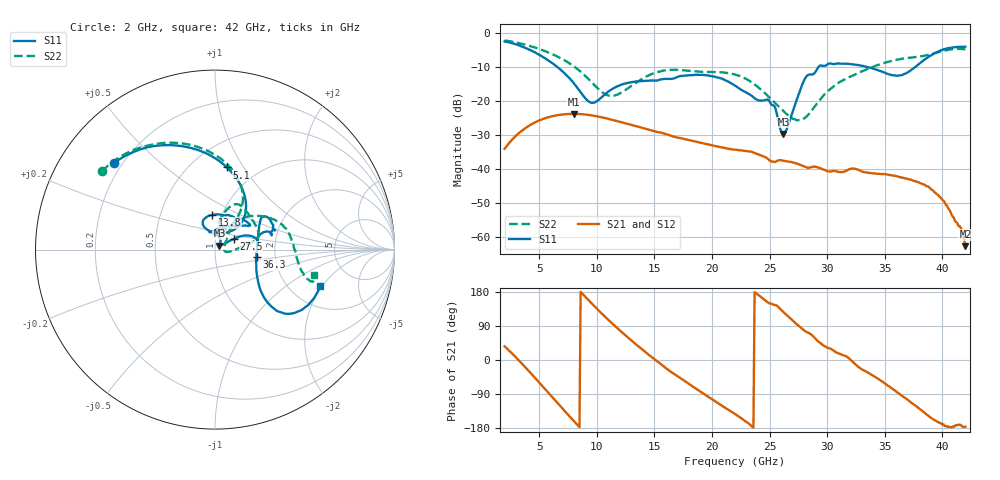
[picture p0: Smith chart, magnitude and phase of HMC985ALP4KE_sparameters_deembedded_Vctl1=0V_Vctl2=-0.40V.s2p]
!s2p File: Measurements: S11, S21, S12, S22
# GHz S dB R 50.0
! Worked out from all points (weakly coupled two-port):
!   401 points, 2 GHz to 42 GHz, reference 50 ohm
!   highest |S21| = -23.91 dB at 8 GHz (marker M1); lowest = -62.8 dB at 42 GHz (marker M2)
!   lowest |S11| = -29.8 dB at 26.2 GHz (marker M3), VSWR 1.07, Z = 52.5 + j2.22 ohm
!   |S11| at or under -10 dB: 6.532 GHz to 29.27 GHz (22.74 GHz wide, 127 % of centre); 33.34 GHz to 37.69 GHz (4.348 GHz wide, 12.2 % of centre)
!   |S22| runs from -25.8 to -2.3 dB; largest |S21 - S12| = 0.00014
!   S11 on the Smith chart (normalised r, x): 2 GHz: 0.17, +0.36; 5.1 GHz: 0.73, +0.85; 13.8 GHz: 0.90, +0.36; 27.5 GHz: 1.22, +0.15; 36.3 GHz: 1.59, -0.14; 42 GHz: 2.90, -1.91
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2  -2.59 139.6  -34.17 35.9  -34.18 36.0  -2.31 145.3
3.5  -4.08 111.7  -28.86 -9.4  -28.86 -9.4  -3.30 121.4
5.1  -6.70 81.7  -25.70 -62.7  -25.70 -62.7  -4.93 97.0
8  -14.86 45.1  -23.91 -160.7  -23.91 -160.8  -9.88 61.0
8.7  -18.00 51.6  -24.00 176.5  -24.00 176.4  -11.80 56.5
9.7  -20.65 86.9  -24.42 144.9  -24.42 144.8  -15.10 55.9
11.2  -16.90 115.7  -25.54 100.3  -25.55 100.3  -18.60 71.9
13.8  -14.26 95.2  -27.87 31.5  -27.88 31.4  -13.87 77.0
15.4  -13.94 73.0  -29.31 -6.9  -29.31 -7.0  -11.47 68.3
19.4  -12.51 34.7  -32.71 -91.5  -32.71 -91.5  -11.55 34.8
22  -15.58 52.2  -34.43 -142.4  -34.44 -142.4  -12.33 14.5
25  -20.23 97.6  -37.62 149.4  -37.62 149.2  -19.16 -0.5
26.2  -29.81 40.9  -37.66 126.7  -37.67 126.7  -23.10 -10.9
27.5  -18.43 29.6  -38.67 90.6  -38.71 90.4  -25.73 0.2
28.1  -13.37 20.7  -39.49 76.0  -39.53 76.1  -25.00 19.0
28.7  -12.32 12.8  -39.51 65.2  -39.51 65.0  -22.73 35.1
31  -9.09 23.4  -40.96 17.4  -40.99 17.1  -14.74 54.3
35.4  -12.27 12.4  -41.88 -69.9  -41.88 -70.5  -8.51 25.5
36.3  -12.57 -10.1  -42.52 -89.9  -42.47 -90.0  -7.83 17.8
39.8  -5.31 -41.3  -48.41 -166.2  -48.29 -165.4  -5.58 -16.5
41.5  -4.18 -23.1  -56.88 -170.7  -56.64 -171.4  -4.77 -17.3
42  -4.14 -19.0  -62.82 -176.2  -63.08 -169.9  -4.92 -14.4
